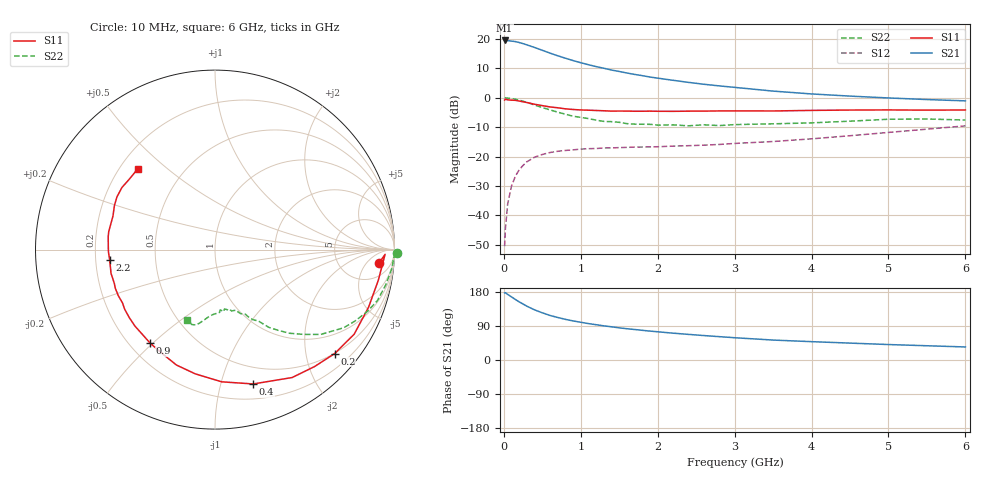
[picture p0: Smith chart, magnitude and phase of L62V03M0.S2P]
!  INFINEON TECHNOLOGIES Small Signal Semiconductors
! BFR380L3 , Si-NPN RF-Transistor in TSLP-3-1
!  Vce=2 V,  Ic=3 mA
! Common Emitter S-Parameters:  07. March 2005
#  GHz  S  MA  R  50
! f  S11  S21  S12  S22
! GHz  Mag  Ang  Mag  Ang  Mag  Ang  Mag  Ang
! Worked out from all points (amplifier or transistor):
!   36 points, 10 MHz to 6 GHz, reference 50 ohm
!   highest |S21| = 19.5 dB at 10 MHz (marker M1)
!   |S21| within 3 dB of that: start of sweep to 463.9 MHz
!   unconditionally stable (mu >= 1): 2.636 GHz to 4.695 GHz
!   at 250 MHz: K = 0.12, MSG = 20.7 dB, |S12| = -23.0 dB
!   at 1.4 GHz: K = 0.64, MSG = 13.2 dB, |S12| = -17.0 dB
!   at 6 GHz: K = 0.93, MSG = 4.3 dB, |S12| = -9.5 dB
!   S11 on the Smith chart (normalised r, x): 10 MHz: 12, -12; 200 MHz: 0.49, -2.59; 400 MHz: 0.33, -1.27; 900 MHz: 0.28, -0.49; 2.2 GHz: 0.26, -0.04; 6 GHz: 0.27, +0.40
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0.01  0.9174 -4.6  9.471 177.0  0.003 84.5  1.015 -1.2
0.02  0.948 -1.6  9.416 177.6  0.0059 91.0  0.9968 -2.5
0.05  0.9259 -10.6  9.425 173.1  0.0157 85.8  0.9914 -5.9
0.1  0.9139 -20.6  9.232 166.5  0.0317 78.8  0.9713 -11.7
0.15  0.9074 -31.3  9.058 159.8  0.0465 73.0  0.9487 -17.4
0.2  0.8832 -41.0  8.732 153.3  0.0598 68.7  0.9163 -22.1
0.3  0.8324 -58.9  7.963 141.9  0.0818 59.8  0.8387 -31.3
0.4  0.7783 -74.1  7.195 132.3  0.0979 52.7  0.7557 -38.7
0.5  0.7376 -87.1  6.443 124.5  0.1088 47.6  0.684 -43.7
0.6  0.701 -99.0  5.764 117.6  0.1175 43.2  0.6242 -48.3
0.7  0.6782 -108.4  5.201 112.2  0.1233 40.7  0.5719 -51.9
0.8  0.6502 -116.7  4.726 107.3  0.1275 38.1  0.5269 -55.3
0.9  0.6344 -124.7  4.307 103.1  0.1305 36.4  0.4874 -57.4
1.1  0.6169 -136.3  3.663 96.0  0.1365 34.8  0.4438 -61.6
1.3  0.603 -146.6  3.189 90.1  0.1403 34.0  0.3975 -64.8
1.6  0.5958 -158.7  2.648 82.5  0.1438 34.1  0.3642 -70.3
2.2  0.5896 -174.5  1.989 70.8  0.151 38.2  0.3469 -77.0
2.8  0.5993 173.1  1.598 61.6  0.1612 44.4  0.3376 -85.1
3.5  0.5984 161.8  1.303 52.6  0.1809 50.5  0.3616 -91.7
4.5  0.6202 151.8  1.071 44.6  0.2269 58.9  0.4012 -99.4
5.5  0.618 140.4  0.936 37.6  0.2934 61.9  0.4371 -107.2
6  0.6223 133.9  0.889 34.4  0.3338 61.5  0.4193 -111.5
